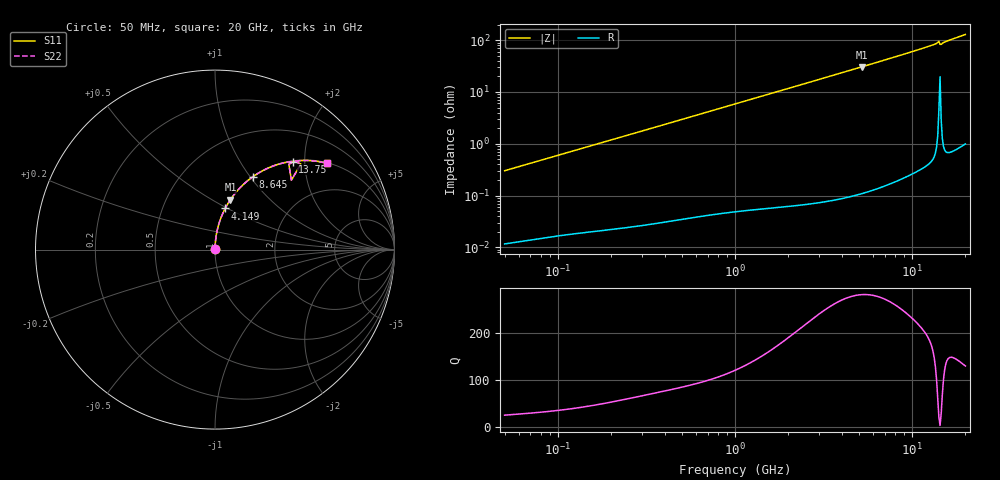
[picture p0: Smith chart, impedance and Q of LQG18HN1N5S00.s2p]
!Murata Part Number: LQG18HN1N5S00
!These Parameters are Measured in Series Mode Connection
!  o--[Z]--o
!Port1  Port2
!  o-------o
!Freq. Start=50[MHz] Stop=20[GHz], 401[Steps]
# Hz S RI R 50
!Freq.(Hz) S11(Real) S11(Imag) S21(Real) S21(Imag) S12(Real) S12(Imag) S22(Real) S22(Imag)
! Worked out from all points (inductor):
!   401 points, 50 MHz to 20 GHz, reference 50 ohm
!   read as one part in series: L = 954 pH near 51.52 MHz
!   highest Q = 282 at 5.195 GHz (marker M1), where L = 936 pH
!   S11 on the Smith chart (normalised r, x): 50 MHz: 1.00, +0.01; 4.149 GHz: 1.00, +0.49; 8.645 GHz: 1.00, +1.03; 13.75 GHz: 1.02, +1.74; 20 GHz: 1.02, +2.58
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5e7  0.000125 0.00301  0.9999 -0.00301  0.9999 -0.00301  0.000125 0.00301
1.364002e8  0.000255 0.00809  0.9997 -0.00809  0.9997 -0.00809  0.000255 0.00809
3.721004e8  0.000773 0.0219  0.9992 -0.0219  0.9992 -0.0219  0.000773 0.0219
6.380365e8  0.00179 0.0374  0.9982 -0.0374  0.9982 -0.0374  0.00179 0.0374
1e9  0.0039 0.0583  0.9961 -0.0583  0.9961 -0.0583  0.0039 0.0583
1.714689e9  0.0105 0.0992  0.9895 -0.0992  0.9895 -0.0992  0.0105 0.0992
2.728004e9  0.0255 0.1555  0.9745 -0.1555  0.9745 -0.1555  0.0255 0.1555
4.149438e9  0.0567 0.2294  0.9433 -0.2294  0.9433 -0.2294  0.0567 0.2294
5.194772e9  0.0862 0.2789  0.9138 -0.2789  0.9138 -0.2789  0.0862 0.2789
6.217679e9  0.1195 0.3226  0.8805 -0.3226  0.8805 -0.3226  0.1195 0.3226
7.442007e9  0.1638 0.3683  0.8362 -0.3683  0.8362 -0.3683  0.1638 0.3683
8.644534e9  0.2108 0.4059  0.7892 -0.4059  0.7892 -0.4059  0.2108 0.4059
1.004137e10  0.2678 0.4406  0.7322 -0.4406  0.7322 -0.4406  0.2678 0.4406
1.166392e10  0.3355 0.4697  0.6645 -0.4697  0.6645 -0.4697  0.3355 0.4697
1.314879e10  0.3999 0.4868  0.6001 -0.4868  0.6001 -0.4868  0.3999 0.4868
1.375312e10  0.4322 0.4904  0.5678 -0.4904  0.5678 -0.4904  0.4322 0.4904
1.396067e10  0.4487 0.4895  0.5513 -0.4895  0.5513 -0.4895  0.4487 0.4895
1.482269e10  0.4341 0.4885  0.5659 -0.4885  0.5659 -0.4885  0.4341 0.4885
1.504638e10  0.4489 0.4925  0.5511 -0.4925  0.5511 -0.4925  0.4489 0.4925
1.573793e10  0.4813 0.4961  0.5187 -0.4961  0.5187 -0.4961  0.4813 0.4961
1.940974e10  0.6069 0.4847  0.3931 -0.4847  0.3931 -0.4847  0.6069 0.4847
2e10  0.6242 0.4805  0.3758 -0.4805  0.3758 -0.4805  0.6242 0.4805
